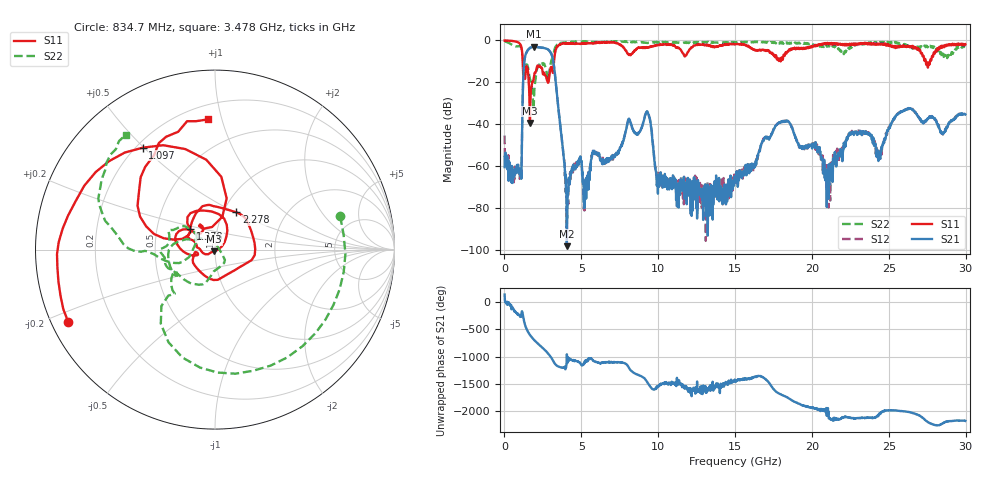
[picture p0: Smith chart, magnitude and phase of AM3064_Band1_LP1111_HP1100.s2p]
# Hz S DB R 50.0
!freq dBS11 angS11 dBS21 angS21 dBS12 angS12 dBS22 angS22
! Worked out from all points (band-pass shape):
!   1600 points, 10 MHz to 29.98 GHz, reference 50 ohm
!   highest |S21| = -3.05 dB at 1.903 GHz (marker M1); lowest = -98.1 dB at 4.059 GHz (marker M2)
!   |S21| within 3 dB of the highest: 1.417 GHz to 3.021 GHz (1.604 GHz wide, 72.3 % of centre)
!   lowest |S11| = -39.4 dB at 1.659 GHz (marker M3), VSWR 1.02, Z = 49.5 - j0.952 ohm
!   |S11| at or under -10 dB: 1.186 GHz to 3.223 GHz (2.037 GHz wide, 92.4 % of centre); 17.96524 GHz to 17.9701 GHz (4.864 MHz wide, 0.0271 % of centre); 27.4 GHz to 27.68 GHz (280.5 MHz wide, 1.02 % of centre)
!   |S22| runs from -33.2 to -0.2 dB; largest |S21 - S12| = 0.011
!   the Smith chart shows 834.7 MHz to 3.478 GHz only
!   S11 on the Smith chart (normalised r, x): 834.7 MHz: 0.05, -0.23; 1.097 GHz: 0.23, +0.50; 1.378 GHz: 0.74, +0.17; 2.278 GHz: 1.15, +0.51; 3.478 GHz: 0.29, +0.91
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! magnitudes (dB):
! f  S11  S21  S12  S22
! 10 MHz  -0.1  -60.4  -45.3  -0.2
! 834.7 MHz  -0.8  -60.3  -60.1  -2.8
! 1.097 GHz  -3.1  -66.0  -66.3  -3.6
! 1.378 GHz  -15.0  -6.8  -6.8  -11.8
! 1.659 GHz  -39.4  -3.6  -3.6  -18.5
! 1.903 GHz  -18.1  -3.1  -3.0  -31.6
! 2.278 GHz  -12.4  -3.3  -3.3  -11.4
! 3.065 GHz  -12.9  -6.7  -6.7  -9.3
! 3.478 GHz  -2.8  -30.3  -30.2  -1.8
! 4.059 GHz  -1.3  -98.1  -79.0  -1.0
! 5.015 GHz  -1.4  -57.5  -58.3  -0.6
! 9.288 GHz  -3.5  -34.1  -34.0  -1.3
! 10 GHz  -2.2  -65.3  -67.5  -0.9
! 13.24 GHz  -2.3  -76.1  -81.6  -0.7
! 15 GHz  -1.7  -66.4  -67.9  -1.3
! 17.97 GHz  -10.0  -39.1  -38.7  -1.1
! 19.99 GHz  -3.4  -50.3  -49.3  -1.8
! 21 GHz  -1.2  -75.0  -64.5  -2.9
! 22.5 GHz  -2.3  -44.2  -43.9  -2.9
! 24.34 GHz  -2.0  -54.3  -53.2  -1.2
! 25 GHz  -2.0  -42.1  -41.3  -1.0
! 29.98 GHz  -1.8  -35.3  -35.4  -2.9
